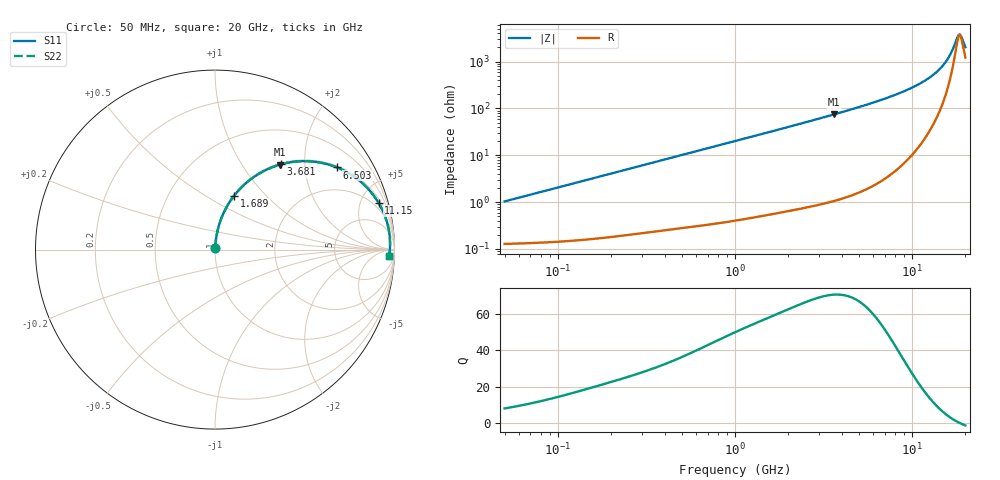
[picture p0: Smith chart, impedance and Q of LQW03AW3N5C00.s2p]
!Murata Part Number: LQW03AW3N5C00
!These Parameters are Measured in Series Mode Connection
!  o--[Z]--o
!Port1  Port2
!  o-------o
!Freq. Start=50[MHz] Stop=20[GHz], 401[Steps]
# Hz S RI R 50
!Freq.(Hz) S11(Real) S11(Imag) S21(Real) S21(Imag) S12(Real) S12(Imag) S22(Real) S22(Imag)
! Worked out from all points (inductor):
!   401 points, 50 MHz to 20 GHz, reference 50 ohm
!   read as one part in series: L = 3.27 nH near 51.52 MHz
!   highest Q = 70.6 at 3.626 GHz (marker M1), where L = 3.28 nH
!   self-resonance near 18.56 GHz
!   S11 on the Smith chart (normalised r, x): 50 MHz: 1.00, +0.02; 1.689 GHz: 1.01, +0.68; 3.681 GHz: 1.02, +1.52; 6.503 GHz: 1.05, +2.93; 11.15 GHz: 1.34, +6.88; 20 GHz: 25, -32
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5e7  0.00139 0.0103  0.9986 -0.0103  0.9986 -0.0103  0.00139 0.0103
1.364002e8  0.00233 0.0278  0.9977 -0.0278  0.9977 -0.0278  0.00233 0.0278
3.721004e8  0.00798 0.0744  0.992 -0.0744  0.992 -0.0744  0.00798 0.0744
1e9  0.0422 0.1912  0.9578 -0.1912  0.9578 -0.1912  0.0422 0.1912
1.689197e9  0.107 0.3009  0.893 -0.3009  0.893 -0.3009  0.107 0.3009
2.728004e9  0.2374 0.4182  0.7626 -0.4182  0.7626 -0.4182  0.2374 0.4182
3.626126e9  0.3597 0.4729  0.6403 -0.4729  0.6403 -0.4729  0.3597 0.4729
3.680849e9  0.367 0.475  0.633 -0.475  0.633 -0.475  0.367 0.475
4.966507e9  0.5277 0.4918  0.4723 -0.4918  0.4723 -0.4918  0.5277 0.4918
6.503449e9  0.6792 0.4579  0.3208 -0.4579  0.3208 -0.4579  0.6792 0.4579
7.442007e9  0.7498 0.4228  0.2502 -0.4228  0.2502 -0.4228  0.7498 0.4228
9.316812e9  0.8505 0.3413  0.1495 -0.3413  0.1495 -0.3413  0.8505 0.3413
1.115139e10  0.9114 0.2607  0.0886 -0.2607  0.0886 -0.2607  0.9114 0.2607
1.314879e10  0.9497 0.1793  0.0503 -0.1793  0.0503 -0.1793  0.9497 0.1793
1.504638e10  0.9683 0.1098  0.0317 -0.1098  0.0317 -0.1098  0.9683 0.1098
1.573793e10  0.9719 0.0865  0.0281 -0.0865  0.0281 -0.0865  0.9719 0.0865
1.646126e10  0.9742 0.0631  0.0258 -0.0631  0.0258 -0.0631  0.9742 0.0631
1.774144e10  0.9753 0.0242  0.0247 -0.0242  0.0247 -0.0242  0.9753 0.0242
1.828096e10  0.9748 0.00868  0.0252 -0.00868  0.0252 -0.00868  0.9748 0.00868
1.855685e10  0.9743 0.000973  0.0257 -0.000973  0.0257 -0.000973  0.9743 0.000973
1.88369e10  0.9737 -0.00672  0.0263 0.00672  0.0263 0.00672  0.9737 -0.00672
2e10  0.9699 -0.0372  0.0301 0.0372  0.0301 0.0372  0.9699 -0.0372
